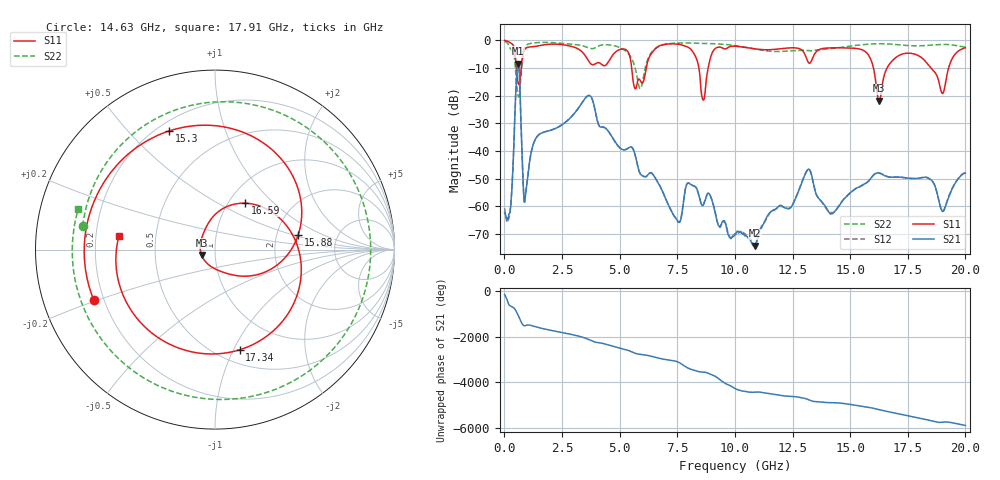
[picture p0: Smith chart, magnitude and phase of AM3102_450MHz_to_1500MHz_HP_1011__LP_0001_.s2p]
!Agilent Technologies,E8364B,MY43040894,A.07.50.67
!Agilent E8364B: A.07.50.67
!Date: Thursday, January 11, 2018 06:23:08
!Correction: S11(Full 2 Port(1,2))
!S21(Full 2 Port(1,2))
!S12(Full 2 Port(1,2))
!S22(Full 2 Port(1,2))
!S2P File: Measurements: S11, S21, S12, S22:
# Hz S  dB  R 50
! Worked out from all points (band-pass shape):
!   1601 points, 10 MHz to 20 GHz, reference 50 ohm
!   highest |S21| = -8.39 dB at 597.2 MHz (marker M1); lowest = -74.2 dB at 10.85 GHz (marker M2)
!   |S21| within 3 dB of the highest: 546.4 MHz to 646.8 MHz (100.4 MHz wide, 16.8 % of centre)
!   lowest |S11| = -21.8 dB at 16.25 GHz (marker M3), VSWR 1.18, Z = 43 - j2.62 ohm
!   |S11| at or under -10 dB: 5.522 GHz to 6.156 GHz (634.1 MHz wide, 10.9 % of centre); 16.01 GHz to 16.6 GHz (591.9 MHz wide, 3.63 % of centre); 18.5 GHz to 19.27 GHz (767.8 MHz wide, 4.06 % of centre)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
!   |S22| runs from -20.6 to -0.4 dB; largest |S21 - S12| = 0.0034
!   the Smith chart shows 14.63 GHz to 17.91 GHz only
!   S11 on the Smith chart (normalised r, x): 14.63 GHz: 0.16, -0.19; 15.3 GHz: 0.25, +0.66; 15.88 GHz: 2.64, +0.54; 16.59 GHz: 1.19, +0.68; 17.34 GHz: 0.63, -1.06; 17.91 GHz: 0.30, +0.07
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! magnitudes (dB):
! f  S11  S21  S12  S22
! 10 MHz  -0.1  -62.3  -60.8  -0.4
! 259.9 MHz  -0.9  -61.2  -60.7  -3.0
! 597.2 MHz  -15.5  -8.4  -8.4  -20.0
! 909.5 MHz  -3.0  -56.3  -56.3  -2.1
! 1.397 GHz  -2.1  -35.1  -35.1  -0.9
! 3.346 GHz  -4.0  -22.9  -22.9  -1.9
! 5.895 GHz  -14.5  -48.2  -48.3  -17.5
! 6.682 GHz  -2.2  -51.6  -51.7  -2.3
! 8.618 GHz  -21.6  -59.7  -59.5  -1.1
! 10.01 GHz  -2.1  -70.0  -70.1  -1.9
! 10.85 GHz  -3.1  -74.2  -74.3  -3.1
! 13.34 GHz  -7.1  -49.2  -49.1  -3.8
! 14.63 GHz  -2.7  -58.5  -58.4  -2.5
! 15.3 GHz  -3.0  -53.3  -53.4  -1.8
! 15.88 GHz  -6.6  -50.1  -50.1  -1.3
! 16.25 GHz  -21.8  -47.9  -48.0  -1.2
! 16.59 GHz  -10.2  -49.3  -49.2  -1.3
! 16.68 GHz  -9.0  -49.5  -49.4  -1.3
! 17.34 GHz  -4.8  -49.6  -49.7  -1.8
! 17.91 GHz  -5.4  -50.0  -50.0  -2.0
! 19 GHz  -19.2  -61.8  -61.9  -1.5
! 20 GHz  -2.7  -48.0  -47.9  -2.4
